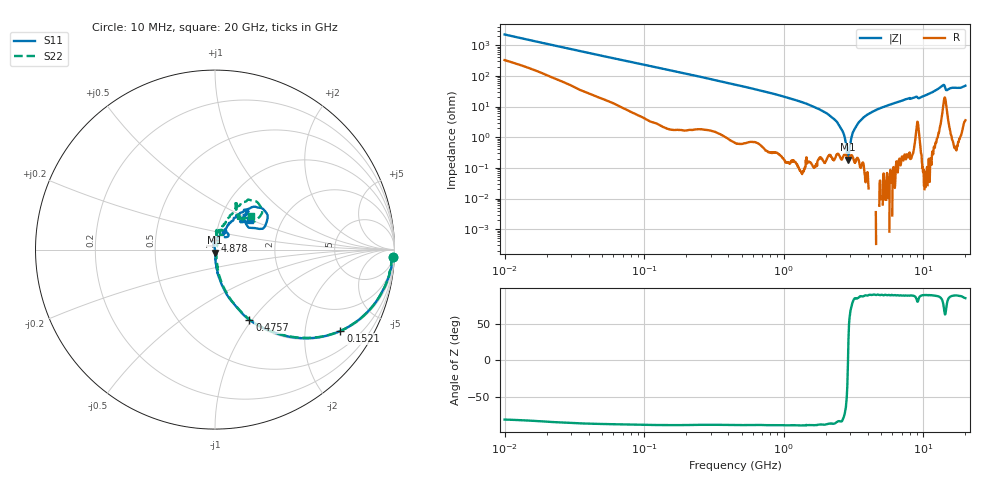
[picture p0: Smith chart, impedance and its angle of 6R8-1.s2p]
!Keysight Technologies,P5008B,MY61100088,A.16.20.02
!Date: Monday, May 27, 2024 16:35:31
!Correction: S11(C* 2-Port  )
!S21(C* 2-Port  )
!S12(C* 2-Port  )
!S22(C* 2-Port  )
!S2P File: Measurements: S11, S21, S12, S22:Log Frequency Sweep
# Hz S  dB  R 50
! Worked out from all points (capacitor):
!   1601 points, 10 MHz to 20 GHz, reference 50 ohm
!   read as one part in series: C = 7.22 pF near 10.39 MHz
!   lowest |Z| = 184 mohm at 2.893 GHz (marker M1)
!   series resonance near 2.884 GHz, so ESL is about 420 pH
!   S11 on the Smith chart (normalised r, x): 10 MHz: 5, -45; 152.1 MHz: 1.03, -3.06; 475.7 MHz: 1.00, -0.97; 4.878 GHz: 0.99, +0.10; 20 GHz: 1.39, +0.49
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1e7  -0.05 -2.5  -27.04 79.1  -27.05 79.1  -0.07 -2.5
3.555162e7  -0.18 -8.9  -16.10 78.0  -16.11 78.0  -0.18 -9.0
1.263918e8  -1.19 -28.5  -6.46 60.7  -6.47 60.7  -1.18 -28.5
1.521183e8  -1.59 -33.0  -5.33 56.4  -5.34 56.4  -1.58 -32.9
4.472136e8  -6.79 -62.5  -1.08 27.0  -1.09 27.0  -6.78 -62.2
4.75703e8  -7.20 -63.9  -0.97 25.6  -0.98 25.6  -7.19 -63.6
1.589917e9  -19.21 -84.9  -0.05 5.5  -0.06 5.5  -19.10 -81.9
2.347211e9  -26.39 -87.5  -0.00 1.3  -0.01 1.3  -26.11 -79.7
2.89288e9  -35.43 -89.3  0.01 -1.0  -0.00 -1.0  -35.22 -67.0
3.004939e9  -37.60 -81.4  0.01 -1.4  -0.00 -1.4  -37.25 -54.4
3.211587e9  -50.21 -115.7  0.01 -2.1  -0.00 -2.1  -42.03 2.6
3.257685e9  -52.43 -123.0  0.01 -2.3  -0.00 -2.3  -41.36 11.4
3.399988e9  -44.88 97.7  0.01 -2.8  -0.00 -2.8  -36.92 41.8
3.53169e9  -40.04 108.8  0.01 -3.2  -0.00 -3.2  -35.20 54.9
3.774562e9  -33.74 104.1  0.01 -4.0  -0.00 -4.0  -31.19 62.9
4.878388e9  -25.88 90.4  0.01 -7.1  -0.00 -7.1  -25.47 70.9
5.652411e9  -23.55 79.5  -0.00 -9.0  -0.01 -9.0  -23.60 81.1
7.697294e9  -18.79 61.1  -0.03 -14.2  -0.04 -14.2  -18.99 83.6
9.577292e9  -20.52 62.4  -0.04 -17.5  -0.05 -17.5  -20.32 75.1
1.361179e10  -9.50 44.2  -0.89 -31.1  -0.90 -31.1  -9.45 55.4
1.468675e10  -12.94 40.2  -0.82 -23.6  -0.83 -23.6  -12.84 50.5
2e10  -11.79 39.8  -0.55 -40.0  -0.56 -40.0  -11.35 43.0
